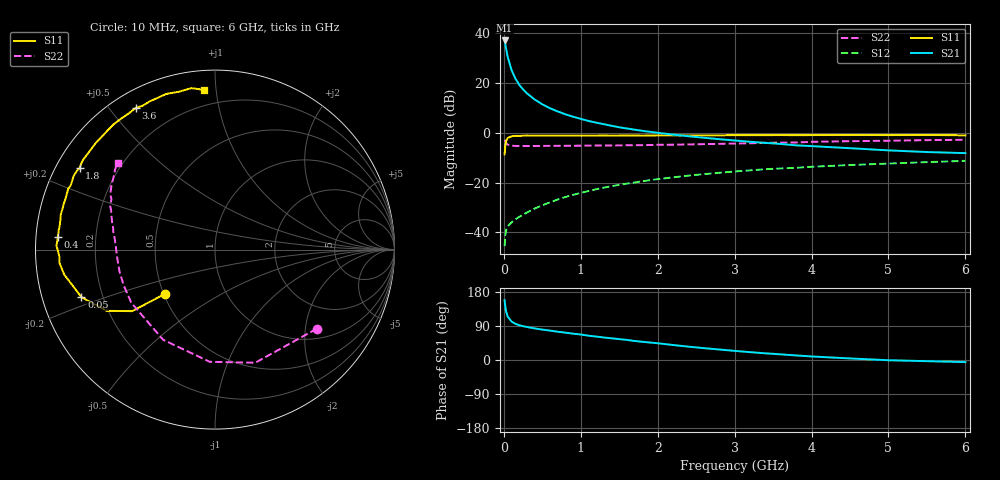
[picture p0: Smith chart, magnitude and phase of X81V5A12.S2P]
! SIEMENS Small Signal Semiconductors
! BFP136W
! Si NPN RF Bipolar Junction Transistor in SOT343
! VCE = 1.5 V  IC = 120 mA
! Common Emitter S-Parameters:  September  1994
# GHz  S  MA  R  50
!  f  S11  S21  S12  S22
! GHz  MAG  ANG  MAG  ANG  MAG  ANG  MAG  ANG
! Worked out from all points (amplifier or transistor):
!   40 points, 10 MHz to 6 GHz, reference 50 ohm
!   highest |S21| = 37.1 dB at 10 MHz (marker M1)
!   |S21| within 3 dB of that: start of sweep to 27.88 MHz
!   unconditionally stable (mu >= 1): 422.4 MHz to 3.269 GHz; 3.749 GHz to 3.87 GHz; 5.888 GHz to end of sweep
!   at 200 MHz: K = 0.77, MSG = 26.5 dB, |S12| = -33.7 dB
!   at 1.5 GHz: K = 1.12, MAG = 9.4 dB, |S12| = -20.9 dB
!   at 6 GHz: K = 1.01, MAG = 0.9 dB, |S12| = -11.2 dB
!   S11 on the Smith chart (normalised r, x): 10 MHz: 0.51, -0.29; 50 MHz: 0.12, -0.17; 400 MHz: 0.06, +0.04; 1.8 GHz: 0.07, +0.28; 3.6 GHz: 0.07, +0.58; 6 GHz: 0.11, +0.93
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0.01  0.3704 -138.4  71.81 157.6  0.0053 66.9  0.718 -37.9
0.02  0.5751 -143.4  59.65 139.8  0.0089 53.3  0.6691 -70.4
0.03  0.6931 -150.5  48.69 128.0  0.0112 45.2  0.6257 -92.7
0.05  0.7898 -160.4  33.67 114.6  0.0133 37.3  0.5795 -119.9
0.1  0.8515 -170.6  18.24 101.4  0.016 37.2  0.5526 -147.5
0.15  0.8701 -175.2  12.35 95.5  0.0183 41.0  0.5462 -158.2
0.2  0.8681 -177.6  9.251 91.9  0.0206 44.5  0.5447 -163.9
0.25  0.8775 180.0  7.455 89.2  0.0227 47.9  0.5457 -167.5
0.3  0.8832 178.6  6.232 87.2  0.0251 50.7  0.5447 -169.9
0.4  0.8785 175.3  4.691 83.4  0.0302 55.1  0.5459 -173.3
0.5  0.8771 173.0  3.741 80.2  0.0351 58.1  0.5468 -175.6
0.6  0.8756 171.2  3.122 77.6  0.0403 60.0  0.5482 -177.2
0.7  0.8774 168.8  2.694 74.6  0.0459 61.6  0.5493 -178.4
0.9  0.8795 165.3  2.11 69.5  0.0569 62.6  0.5513 179.2
1.1  0.88 161.2  1.734 64.1  0.0677 62.6  0.5546 177.6
1.8  0.8805 148.9  1.099 48.1  0.1067 59.0  0.5666 171.7
2.2  0.8881 142.3  0.923 39.6  0.1278 55.6  0.5784 168.5
3.2  0.8979 125.4  0.663 20.7  0.1765 45.4  0.6181 159.4
3.6  0.9043 119.3  0.599 14.9  0.1929 41.3  0.6364 155.9
4.5  0.9086 107.4  0.492 4.1  0.2259 32.6  0.6808 147.8
5.5  0.9091 98.3  0.412 -3.1  0.2584 24.6  0.7141 141.2
6  0.8926 94.1  0.392 -5.6  0.2744 20.2  0.7261 138.3
